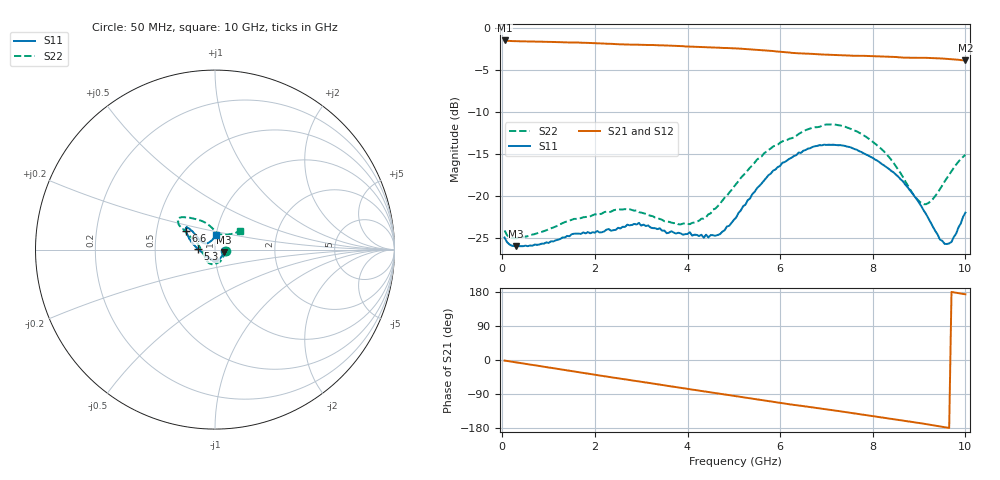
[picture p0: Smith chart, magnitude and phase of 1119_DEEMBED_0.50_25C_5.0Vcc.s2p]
!Hittite Microwave Corp.
!Digital Attenuator/PhaseShifter Rev 1.4.0
!Filename: C:\DATA\DATA\1119_DEEMBED_0.50_25C_5.0Vcc.s2p
!VNA ID: Agilent Technologies,N5224A,MY51441122,A.10.45.03
!Device type:
!2 Port Calibration.
!Temp(C): 25
!Lot Number:
!Serial Number:
!Operator:
!Misc:
!Attenuator:  0.500
# GHZ S DB R 50.0
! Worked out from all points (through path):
!   200 points, 50 MHz to 10 GHz, reference 50 ohm
!   highest |S21| = -1.47 dB at 50 MHz (marker M1); lowest = -3.9 dB at 10 GHz (marker M2)
!   group delay of S21, straight-line fit = 51 ps
!   lowest |S11| = -26.0 dB at 300 MHz (marker M3), VSWR 1.11, Z = 55.1 - j1.49 ohm
!   |S11| at or under -10 dB: start of sweep to end of sweep
!   |S22| runs from -25.0 to -11.5 dB; largest |S21 - S12| = 0.0021
!   S11 on the Smith chart (normalised r, x): 50 MHz: 1.12, -0.02; 5.3 GHz: 0.83, +0.00; 6.6 GHz: 0.71, +0.15; 10 GHz: 1.00, +0.16
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0.05  -24.94 -10.2  -1.47 -1.6  -1.47 -1.6  -24.10 -9.6
0.3  -25.97 -15.6  -1.56 -6.2  -1.56 -6.2  -25.03 -16.9
1.75  -24.33 -73.7  -1.74 -34.1  -1.74 -34.1  -22.53 -75.2
2.65  -23.67 -86.7  -1.95 -51.0  -1.95 -51.1  -21.55 -107.2
2.95  -23.20 -91.9  -1.98 -56.4  -1.98 -56.5  -21.92 -118.5
3.4  -23.84 -98.8  -2.04 -64.9  -2.04 -65.0  -22.73 -133.2
3.85  -24.44 -105.0  -2.14 -73.4  -2.15 -73.5  -23.38 -148.7
4.35  -24.97 -121.0  -2.26 -82.6  -2.28 -82.7  -22.69 -175.7
4.7  -24.55 -143.5  -2.34 -89.1  -2.36 -89.2  -20.92 167.4
5.05  -22.55 -168.0  -2.42 -95.7  -2.43 -95.7  -18.56 156.7
5.3  -20.49 178.2  -2.50 -100.5  -2.51 -100.5  -16.94 153.6
5.85  -16.97 161.2  -2.73 -110.7  -2.75 -110.8  -14.09 148.2
6.6  -14.35 147.6  -3.05 -123.5  -3.06 -123.5  -12.05 144.7
6.7  -14.15 146.3  -3.07 -125.2  -3.08 -125.2  -11.87 143.6
7.45  -14.12 141.7  -3.26 -138.1  -3.27 -138.1  -11.84 135.0
8.35  -16.78 142.1  -3.40 -154.4  -3.41 -154.4  -15.35 113.2
8.9  -20.03 148.5  -3.53 -164.3  -3.53 -164.3  -20.00 88.0
9.15  -22.14 150.7  -3.54 -169.1  -3.55 -169.2  -20.97 71.2
9.45  -25.18 140.4  -3.60 -175.2  -3.61 -175.3  -19.19 49.9
9.6  -25.71 125.0  -3.66 -178.4  -3.67 -178.4  -17.86 43.0
9.7  -25.46 112.4  -3.70 179.6  -3.71 179.6  -17.05 40.1
10  -21.98 86.0  -3.85 173.3  -3.86 173.3  -15.10 36.8
